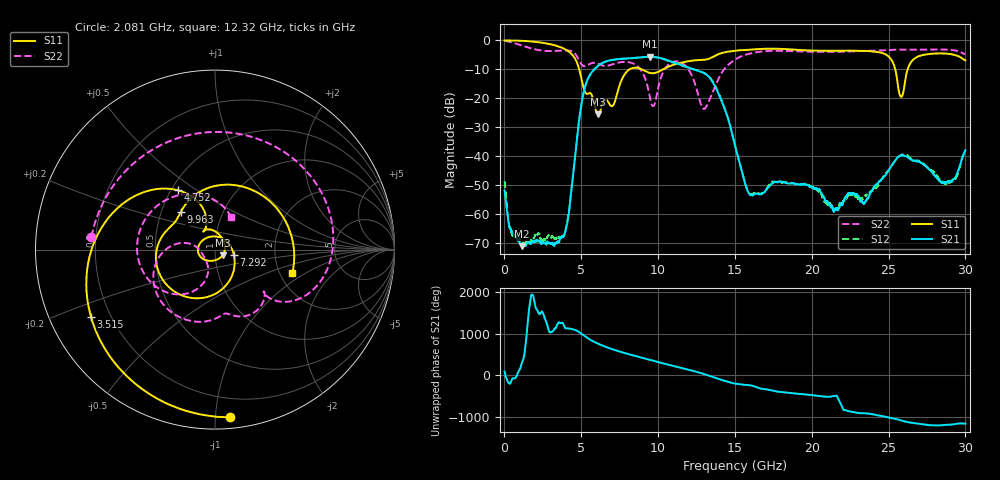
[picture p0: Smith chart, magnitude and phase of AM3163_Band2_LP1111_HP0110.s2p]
!Agilent Technologies,E8364B,MY43040894,A.07.50.67
!Agilent E8364B: A.07.50.67
!Date: Thursday, August 20, 2020 12:07:20
!Correction: S11(Full 2 Port(1,2))
!S21(Full 2 Port(1,2))
!S12(Full 2 Port(1,2))
!S22(Full 2 Port(1,2))
!S2P File: Measurements: S11, S21, S12, S22:
# Hz S  dB  R 50
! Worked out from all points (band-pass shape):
!   3201 points, 10 MHz to 30 GHz, reference 50 ohm
!   highest |S21| = -5.67 dB at 9.457 GHz (marker M1); lowest = -71.2 dB at 1.125 GHz (marker M2)
!   |S21| within 3 dB of the highest: 6.12 GHz to 11.58 GHz (5.459 GHz wide, 61.7 % of centre)
!   lowest |S11| = -25.6 dB at 6.102 GHz (marker M3), VSWR 1.11, Z = 54.4 - j3.36 ohm
!   |S11| at or under -10 dB: 4.864 GHz to 8.144 GHz (3.28 GHz wide, 50.4 % of centre); 8.942 GHz to 10.33 GHz (1.386 GHz wide, 14.4 % of centre); 25.43 GHz to 26.24 GHz (804.6 MHz wide, 3.11 % of centre)
!   |S22| runs from -23.7 to -0.1 dB; largest |S21 - S12| = 0.012
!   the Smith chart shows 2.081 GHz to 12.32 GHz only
!   S11 on the Smith chart (normalised r, x): 2.081 GHz: 0.07, -1.09; 3.515 GHz: 0.13, -0.25; 4.752 GHz: 0.54, +0.42; 7.292 GHz: 1.23, -0.07; 9.963 GHz: 0.63, +0.28; 12.32 GHz: 2.34, -0.77
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1e7  -0.01 -2.9  -51.98 89.8  -48.62 12.1  -0.14 -6.9
1.125253e9  -0.14 -45.3  -71.19 -68.9  -70.15 -15.3  -1.75 -106.3
2.081184e9  -0.55 -85.0  -69.40 159.2  -66.93 -62.0  -3.20 174.1
3.515081e9  -2.09 -151.4  -69.65 -166.4  -68.26 78.4  -3.57 64.4
4.752169e9  -8.15 122.2  -32.33 -15.2  -32.37 -15.7  -5.83 -34.4
5.014581e9  -13.36 105.2  -21.87 -78.8  -21.89 -79.1  -8.27 -41.9
6.101719e9  -25.55 -35.7  -8.75 40.0  -8.79 39.8  -8.05 -70.1
7.291947e9  -19.23 -15.8  -6.52 -125.1  -6.59 -125.0  -7.82 -99.0
8.529034e9  -9.44 -158.9  -6.04 104.3  -6.04 104.5  -8.39 -154.5
9.45685e9  -11.22 150.2  -5.67 13.2  -5.66 13.0  -19.53 171.7
9.962931e9  -10.97 132.7  -5.91 -37.1  -5.94 -37.6  -17.46 -106.8
1.000979e10  -10.86 130.6  -5.96 -41.7  -5.99 -42.3  -16.25 -106.4
1.232464e10  -6.93 -16.9  -10.02 101.3  -9.98 102.7  -13.85 63.3
1.303691e10  -6.68 -51.2  -11.44 25.0  -11.38 26.5  -23.61 -114.0
1.5005e10  -3.56 -132.7  -36.40 160.4  -36.38 159.5  -6.69 -112.2
1.600779e10  -3.20 -174.4  -53.49 117.2  -53.20 118.0  -4.51 -172.5
1.787279e10  -2.90 98.1  -48.79 -37.6  -49.22 -37.2  -3.58 92.0
2.000958e10  -3.51 -9.9  -50.67 -119.4  -50.78 -122.1  -3.94 -9.6
2.231506e10  -3.55 -100.2  -53.48 -136.9  -53.81 -141.8  -3.85 -93.8
2.500479e10  -5.57 157.5  -44.93 62.6  -44.79 65.7  -3.36 -167.6
2.582014e10  -19.52 171.4  -39.79 -9.2  -39.60 -7.4  -3.22 170.3
3e10  -6.90 51.8  -37.99 -86.8  -38.23 -91.1  -4.78 55.1
